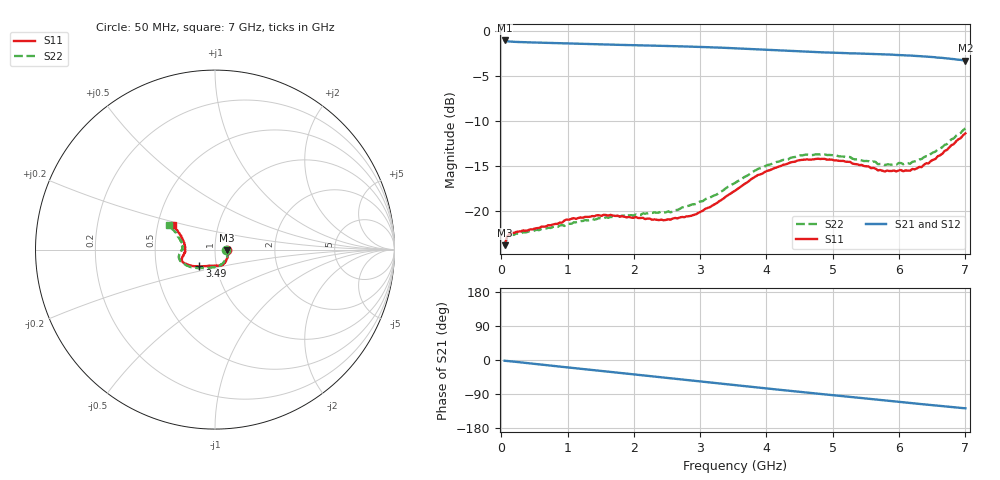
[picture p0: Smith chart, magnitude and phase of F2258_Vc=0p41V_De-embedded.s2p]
! Integrated Device Technology
! Corporate Headquarters
! 6024 Silver Creek Valley Road
! San Jose, CA 95138  USA
! Phone:  1-408-284-8200
! Toll Free:  1-800-223-1366
! Webpage:  http://www.idt.com/
! Timing and RF Division
! 515 Groton Road, Suite 102
! Westford, MA 01886-6024
! Device:  F2258
! Description: Voltage Variable RF Attenuator
! Frequency:  50.0 -  6000.00 MHz
! Package:  3x3 mm Thin QFN Plastic Package: 16 pin
! Ports:  2 RF, 2 DC
!  Pin  1  = NC
!  Pin  2  = NC
!  Pin  3  = RF2  = Port 2
!  Pin  4  = GND
!  Pin  5  = Vdd
!  Pin  6  = NC
!  Pin  7  = VCTRL
!  Pin  8  = NC
!  Pin  9  = GND
!  Pin 10  = RF1  = Port 1
!  Pin 11  = NC
!  Pin 12  = NC
!  Pin 13  = NC
!  Pin 14  = NC
!  Pin 15  = NC
!  Pin 16  = NC
! Vcntrl:  0.410 Volts
! Vdd:  +3.300 Volts
! Current:  1.094 mA
! Data:  The device was measured on a the F2258 evaluation board which has
!  individual transmission lines to the RF pins.  Data was collected
!  using a calibrated network analyzer.  The evaluation board was
!  de-embedded using a TRL calibration technique.
!  The reference plane is the edge of the package pin.
! Misc:  SN 10
!  Action Tracker AT0285
! Date Measured:  2014-12-10
! Date:  2016-01-13  MJV
! Note:
!  Integrated Device Technology supplies this data as a sample of measured
!  data at the package pin for this product.  Your particular data for this
!  product may vary.
!  Data was taken at 25 degrees C.
!  Integrated Device Technology reserves the right to change this data at anytime.
!Freq_(GHz)  S11M_(dB)  S11P_(deg)  S21M_(dB)  S21P_(deg)  S12M_(dB)  S12P_(deg)  S22M_(dB)  S22P_(deg)
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# GHz S dB R 50
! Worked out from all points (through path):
!   201 points, 50 MHz to 7 GHz, reference 50 ohm
!   highest |S21| = -1.03 dB at 50 MHz (marker M1); lowest = -3.3 dB at 7 GHz (marker M2)
!   group delay of S21, straight-line fit = 50.5 ps
!   lowest |S11| = -23.8 dB at 50 MHz (marker M3), VSWR 1.14, Z = 56.9 - j0.424 ohm
!   |S11| at or under -10 dB: start of sweep to end of sweep
!   |S22| runs from -23.9 to -10.8 dB; largest |S21 - S12| = 0.00049
!   S11 on the Smith chart (normalised r, x): 50 MHz: 1.14, -0.01; 3.49 GHz: 0.83, -0.16; 7 GHz: 0.60, +0.18
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0.05  -23.84 -3.3  -1.03 -2.0  -1.03 -2.0  -23.93 -3.1
0.08475  -22.90 -5.4  -1.11 -2.5  -1.11 -2.5  -23.02 -5.2
0.15425  -22.44 -8.5  -1.16 -3.6  -1.16 -3.7  -22.65 -9.0
0.71025  -21.59 -34.4  -1.30 -14.1  -1.30 -14.1  -21.88 -37.0
0.98825  -20.96 -47.7  -1.35 -19.4  -1.35 -19.4  -21.46 -52.5
1.2315  -20.77 -55.7  -1.40 -23.8  -1.40 -23.8  -21.13 -61.4
1.6485  -20.44 -67.0  -1.49 -31.4  -1.49 -31.4  -20.68 -74.5
2.37825  -21.03 -87.5  -1.62 -44.8  -1.62 -44.8  -20.18 -92.6
2.552  -20.98 -93.4  -1.65 -48.0  -1.65 -48.0  -20.16 -97.9
2.93425  -20.39 -110.1  -1.73 -55.1  -1.73 -55.1  -19.24 -111.4
3.49025  -17.91 -133.2  -1.89 -65.6  -1.88 -65.6  -17.03 -132.8
3.525  -17.76 -134.1  -1.90 -66.2  -1.90 -66.2  -16.90 -134.3
4.0115  -15.55 -148.6  -2.07 -75.2  -2.08 -75.2  -14.90 -150.0
4.46325  -14.41 -157.4  -2.24 -83.4  -2.24 -83.4  -13.88 -161.2
4.7065  -14.27 -160.7  -2.31 -87.7  -2.31 -87.7  -13.78 -165.5
5.2625  -14.55 -167.5  -2.46 -97.4  -2.46 -97.4  -14.01 -173.7
5.6795  -15.49 -174.0  -2.54 -104.6  -2.55 -104.6  -14.80 -179.2
5.85325  -15.57 -178.2  -2.60 -107.8  -2.60 -107.8  -14.83 176.1
6.166  -15.53 173.8  -2.71 -113.4  -2.71 -113.4  -14.75 170.1
6.33975  -15.13 167.3  -2.79 -116.5  -2.79 -116.5  -14.23 165.7
6.722  -13.21 155.1  -3.02 -123.1  -3.02 -123.1  -12.56 156.6
7  -11.37 149.3  -3.27 -127.4  -3.27 -127.4  -10.81 151.6
